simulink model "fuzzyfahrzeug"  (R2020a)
settings: Solver=ode45  StartTime=0.0  StopTime=200  MaxStep=0.1  RelTol=1e-3  EnableMultiTasking=on
libraries: libregler2 x4

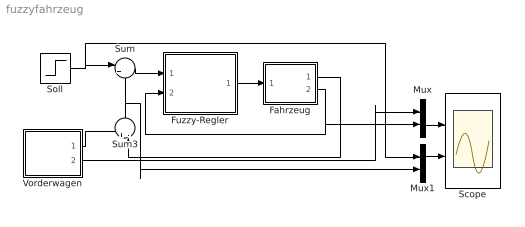
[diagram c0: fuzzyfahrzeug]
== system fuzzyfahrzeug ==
  Fahrzeug : Subsystem  mask{m=1000}
      mask prompts: m "Fahrzeugmasse"
  Fuzzy-Regler : Subsystem
  Mux : Mux  Inputs=2
  Mux1 : Mux  Inputs=2
  Scope : Scope  NumInputPorts=2
  Soll : Step  Time=100  Before=20  After=50  SampleTime=0
  Sum : Sum  Inputs=|+-  SaturateOnIntegerOverflow=on
  Sum3 : Sum  Inputs=+-|  InputSameDT=on  SaturateOnIntegerOverflow=on
  Vorderwagen : Subsystem
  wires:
  Fuzzy-Regler/1(u) -> Fahrzeug/1(F)
  Sum/1 -> Fuzzy-Regler/1(d)
  Fahrzeug/2(vF) -> Fuzzy-Regler/2(v), Mux/2
  Soll/1 -> Sum/1, Mux1/1
  Vorderwagen/1(xV) -> Sum3/1
  Fahrzeug/1(xF) -> Sum3/2
  Sum3/1 -> Sum/2, Mux1/2
  Vorderwagen/2(vV) -> Mux/1
  Mux/1 -> Scope/1
  Mux1/1 -> Scope/2

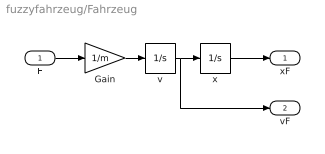
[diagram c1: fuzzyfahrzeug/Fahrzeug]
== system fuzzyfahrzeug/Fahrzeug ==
  F : Inport
  Gain : Gain  Gain=1/m
  v : Integrator
  x : Integrator
  xF : Outport
  vF : Outport  Port=2
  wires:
  F/1 -> Gain/1
  v/1 -> x/1, vF/1
  x/1 -> xF/1
  Gain/1 -> v/1

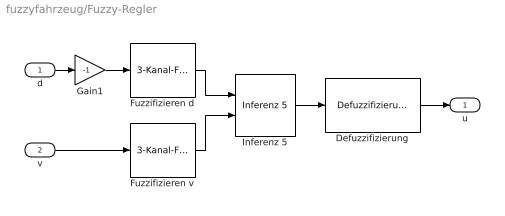
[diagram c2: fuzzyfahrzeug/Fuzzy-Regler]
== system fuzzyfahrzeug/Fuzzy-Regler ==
  d : Inport
  v : Inport  Port=2
  Defuzzifizierung : libregler2/Defuzzifizierung  h=[-3, -1, 0, 1, 3]*1000
  Fuzzifizieren d : libregler2/3-Kanal-Fuzzifizierer  w=10  offset=0
  Fuzzifizieren v : libregler2/3-Kanal-Fuzzifizierer  w=5  offset=20
  Gain1 : Gain  Gain=-1  SaturateOnIntegerOverflow=on
  Inferenz 5 : libregler2/Inferenz 5  M=[3 2 1; 4 3 2; 5 4 3]
  u : Outport
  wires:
  Inferenz 5/1 -> Defuzzifizierung/1
  Defuzzifizierung/1 -> u/1
  d/1 -> Gain1/1
  v/1 -> Fuzzifizieren v/1
  Gain1/1 -> Fuzzifizieren d/1
  Fuzzifizieren v/1 -> Inferenz 5/2
  Fuzzifizieren d/1 -> Inferenz 5/1

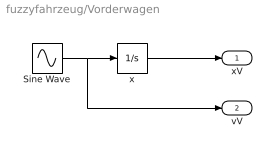
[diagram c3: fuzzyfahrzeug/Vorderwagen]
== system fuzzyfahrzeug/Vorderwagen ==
  Sine Wave : Sin  Bias=20  Frequency=0.1  SampleTime=0
  x : Integrator  InitialCondition=10
  xV : Outport
  vV : Outport  Port=2
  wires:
  x/1 -> xV/1
  Sine Wave/1 -> x/1, vV/1
